(* High speed task. Serial background communication. *)
PROGRAM P_SerialComm_HighSpeed
VAR
	serial_In			AT%I*	: PcComInData;
	serial_Out			AT%Q* 	: PcComOutData;
	KL6_In				AT%I*	: KL6inData5B;
	KL6_Out				AT%Q*	: KL6outData5B;
	
	hSerial				: T_HSERIALCTRL;(* Serial connection control handle *)
	fbSerialLineCtrl	: FB_IEC870_SerialLineCtrl := (	Mode := SERIALLINEMODE_PC_COM_PORT(*SERIALLINEMODE_KL6_5B_STANDARD*),
														Baudrate := 19200,
														NoDatabits := 8,
														Parity := PARITY_EVEN,
														Stopbits := 1,
														Handshake := HANDSHAKE_NONE,
														ContinousMode := FALSE );
END_VAR

fbSerialLineCtrl(	pComIn		:= SEL( fbSerialLineCtrl.Mode = SERIALLINEMODE_KL6_5B_STANDARD, ADR( serial_In ), ADR( KL6_In ) ),
					pComOut		:= SEL( fbSerialLineCtrl.Mode = SERIALLINEMODE_KL6_5B_STANDARD, ADR( serial_Out ), ADR( KL6_Out ) ),
					SizeComIn	:= SEL( fbSerialLineCtrl.Mode = SERIALLINEMODE_KL6_5B_STANDARD, SIZEOF( serial_In ), SIZEOF( KL6_In ) ),
					hSerial		:= hSerial );

END_PROGRAM
